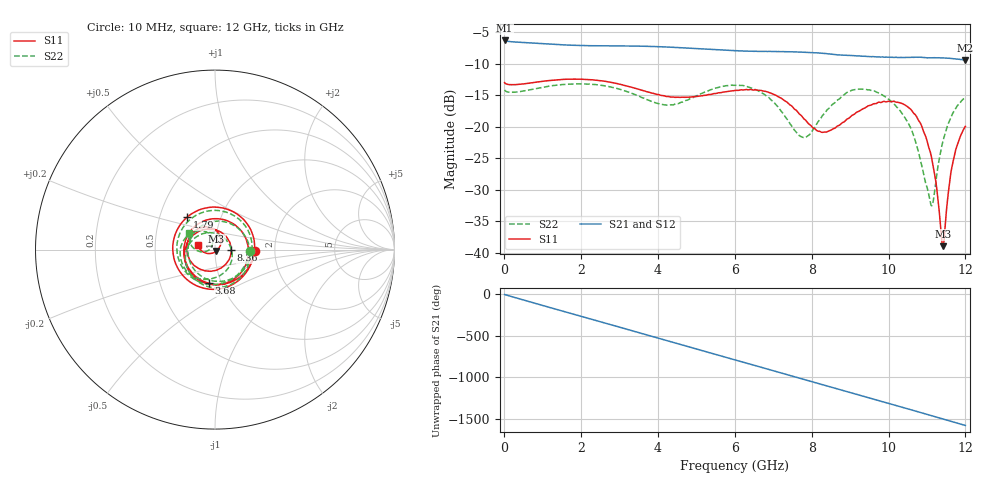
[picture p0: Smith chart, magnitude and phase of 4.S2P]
!Agilent Technologies,E5071C,MY46316741,A.11.02
!Date: Fri Apr 15 15:49:49 2022
!Data & Calibration Information:
!Freq	S11:SOLT2(ON)	S21:SOLT2(ON)	S12:SOLT2(ON)	S22:SOLT2(ON)
!PortZ  Port1:50+j0  Port2:50+j0
!Above PortZ is port z conversion or system Z0 setting when saving the data.
!When reading, reference impedance value at option line is always used.
# Hz S dB R 50
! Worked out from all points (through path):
!   1200 points, 10 MHz to 12 GHz, reference 50 ohm
!   highest |S21| = -6.33 dB at 10 MHz (marker M1); lowest = -9.4 dB at 12 GHz (marker M2)
!   group delay of S21, straight-line fit = 365 ps
!   lowest |S11| = -38.9 dB at 11.41 GHz (marker M3), VSWR 1.02, Z = 50.8 - j0.836 ohm
!   |S11| at or under -10 dB: start of sweep to end of sweep
!   |S22| runs from -32.5 to -13.2 dB; largest |S21 - S12| = 0.0029
!   S11 on the Smith chart (normalised r, x): 10 MHz: 1.57, -0.03; 1.79 GHz: 0.69, +0.26; 3.68 GHz: 0.87, -0.34; 8.36 GHz: 1.20, -0.00; 12 GHz: 0.82, +0.04
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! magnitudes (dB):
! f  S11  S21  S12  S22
! 10 MHz  -13.0  -6.3  -6.3  -14.2
! 1.79 GHz  -12.5  -7.1  -7.1  -13.2
! 2.01 GHz  -12.5  -7.1  -7.1  -13.2
! 3.68 GHz  -14.4  -7.2  -7.3  -15.6
! 4.01 GHz  -14.9  -7.3  -7.3  -16.3
! 6.01 GHz  -14.2  -7.9  -8.0  -13.4
! 7.04 GHz  -14.9  -8.1  -8.1  -16.3
! 7.7 GHz  -18.1  -8.2  -8.2  -21.5
! 8.01 GHz  -20.0  -8.2  -8.2  -20.7
! 8.36 GHz  -20.9  -8.4  -8.4  -17.7
! 9.12 GHz  -18.0  -8.7  -8.7  -14.1
! 10.01 GHz  -16.0  -9.0  -9.0  -15.7
! 10.6 GHz  -17.4  -9.0  -9.0  -20.5
! 10.87 GHz  -20.0  -9.0  -9.0  -26.3
! 11.11 GHz  -24.6  -9.1  -9.1  -32.5
! 11.17 GHz  -26.5  -9.1  -9.1  -31.5
! 11.37 GHz  -37.0  -9.1  -9.1  -23.5
! 11.41 GHz  -38.9  -9.1  -9.1  -22.4
! 11.45 GHz  -37.6  -9.1  -9.1  -21.6
! 11.58 GHz  -29.2  -9.1  -9.1  -19.1
! 11.68 GHz  -25.5  -9.2  -9.2  -17.8
! 12 GHz  -19.9  -9.4  -9.4  -15.3
